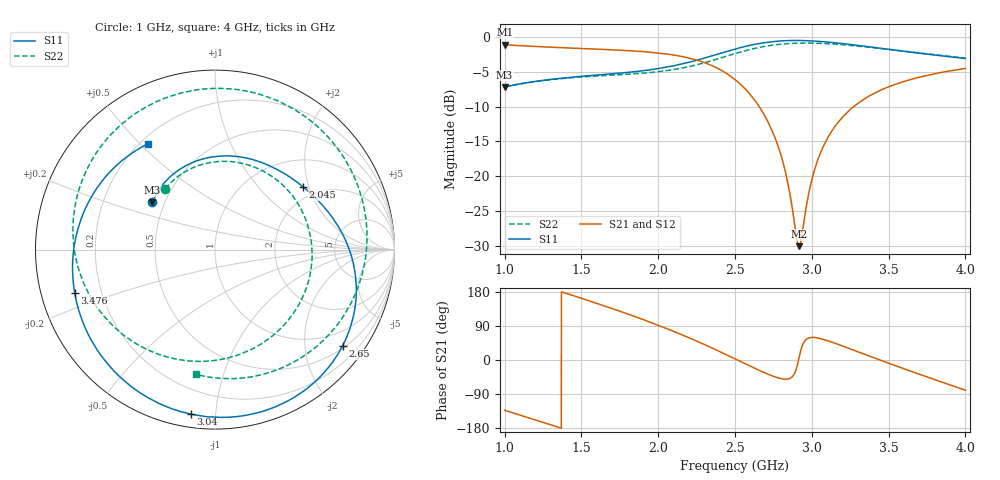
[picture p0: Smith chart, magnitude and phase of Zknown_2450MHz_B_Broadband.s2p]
!Agilent Technologies,N5242A,MY49421279,A.09.90.21
!Agilent N5242A: A.09.90.21
!Date: Monday, January 30, 2023
!Caliblation kit: 85033D 3.5mm Calibration Kit
!DUT Connector Gender Port1: male
!DUT Connector Gender Port2: female
!S2P File: Measurements: S11, S21, S12, S22:
# Hz S  dB  R 50
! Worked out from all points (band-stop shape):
!   3001 points, 1 GHz to 4 GHz, reference 50 ohm
!   highest |S21| = -1.15 dB at 1.001 GHz (marker M1); lowest = -30.0 dB at 2.917 GHz (marker M2)
!   |S21| within 3 dB of the highest: start of sweep to 2.351 GHz
!   lowest |S11| = -7.2 dB at 1 GHz (marker M3), VSWR 2.55, Z = 21.4 + j14 ohm
!   |S11| at or under -10 dB: nowhere
!   |S22| runs from -7.2 to -0.9 dB; largest |S21 - S12| = 0.0049
!   S11 on the Smith chart (normalised r, x): 1 GHz: 0.43, +0.28; 2.045 GHz: 1.67, +1.83; 2.65 GHz: 0.56, -2.89; 3.04 GHz: 0.07, -0.86; 3.476 GHz: 0.10, -0.15; 4 GHz: 0.23, +0.53
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1e9  -7.19 142.9  -1.16 -132.6  -1.16 -132.6  -7.19 129.3
1.001e9  -7.18 142.8  -1.15 -132.7  -1.16 -132.7  -7.18 129.2
1.258e9  -6.23 113.8  -1.46 -165.6  -1.47 -165.5  -6.26 92.6
1.5e9  -5.67 88.1  -1.70 162.9  -1.71 162.9  -5.77 55.9
1.782e9  -5.15 60.1  -1.97 124.2  -1.96 124.3  -5.40 7.2
2e9  -4.56 39.6  -2.34 91.7  -2.32 91.8  -5.01 -37.4
2.045e9  -4.40 35.4  -2.45 84.6  -2.42 84.7  -4.88 -47.6
2.179e9  -3.78 22.5  -2.95 62.4  -2.92 62.4  -4.39 -80.0
2.289e9  -3.13 11.0  -3.62 43.1  -3.58 42.9  -3.80 -108.6
2.391e9  -2.47 -0.9  -4.57 24.1  -4.54 23.8  -3.15 -136.3
2.5e9  -1.78 -15.1  -6.13 3.0  -6.11 2.7  -2.42 -166.5
2.65e9  -1.01 -37.0  -9.75 -25.9  -9.76 -26.3  -1.57 152.7
2.8e9  -0.61 -60.5  -17.01 -49.1  -17.06 -49.4  -1.07 114.2
2.917e9  -0.55 -79.0  -29.99 5.7  -29.96 5.9  -0.93 86.6
3e9  -0.61 -92.0  -20.49 59.7  -20.55 59.3  -0.92 68.4
3.04e9  -0.66 -98.2  -17.57 58.0  -17.63 57.9  -0.94 60.0
3.144e9  -0.86 -114.2  -13.06 45.2  -13.13 45.3  -1.06 39.1
3.248e9  -1.11 -129.7  -10.48 29.7  -10.55 30.0  -1.24 19.6
3.476e9  -1.75 -162.9  -7.39 -4.8  -7.42 -4.3  -1.76 -19.7
3.5e9  -1.81 -166.3  -7.18 -8.4  -7.19 -7.9  -1.82 -23.5
3.745e9  -2.48 158.8  -5.57 -43.9  -5.54 -43.5  -2.44 -61.5
4e9  -3.12 122.4  -4.55 -79.8  -4.50 -79.5  -3.07 -98.5
